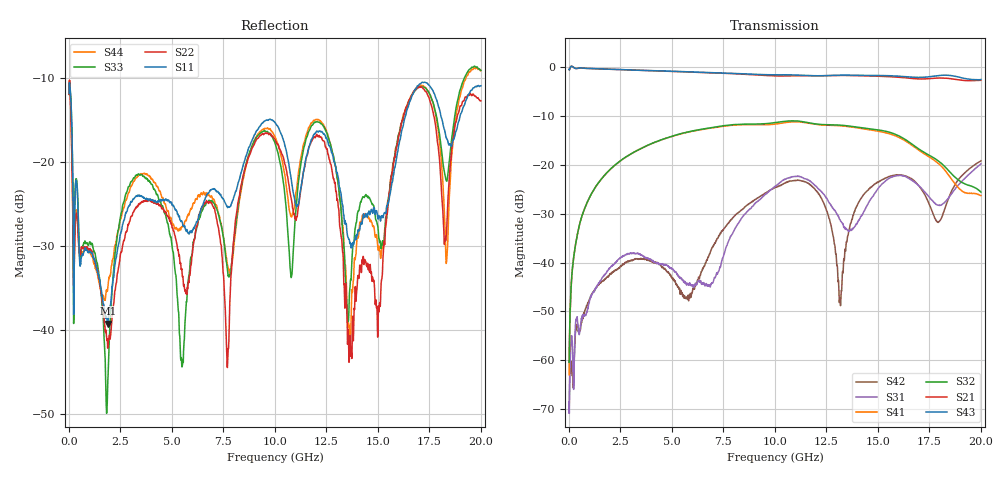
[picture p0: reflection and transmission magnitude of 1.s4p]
!Keysight Technologies,N5225A,MY51451420,A.10.40.12
!Date: Tuesday, October 13, 2015 10:13:44
!Correction: S11(Full 4 Port(1,2,3,4))
!S12(Full 4 Port(1,2,3,4))
!S13(Full 4 Port(1,2,3,4))
!S14(Full 4 Port(1,2,3,4))
!S21(Full 4 Port(1,2,3,4))
!S22(Full 4 Port(1,2,3,4))
!S23(Full 4 Port(1,2,3,4))
!S24(Full 4 Port(1,2,3,4))
!S31(Full 4 Port(1,2,3,4))
!S32(Full 4 Port(1,2,3,4))
!S33(Full 4 Port(1,2,3,4))
!S34(Full 4 Port(1,2,3,4))
!S41(Full 4 Port(1,2,3,4))
!S42(Full 4 Port(1,2,3,4))
!S43(Full 4 Port(1,2,3,4))
!S44(Full 4 Port(1,2,3,4))
!S4P File: Measurements: <S11,S12,S13,S14>,
!<S21,S22,S23,S24>,
!<S31,S32,S33,S34>,
!<S41,S42,S43,S44>:
# Hz S  dB  R 50
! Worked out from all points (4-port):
!   1999 points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, 20 MHz to 20 GHz, reference 50 ohm
!   strongest paths, dB at 20 MHz, 5.01 GHz, 10.01 GHz, 15.01 GHz, 20 GHz:
!     S43: -0.5, -0.9, -1.6, -1.7, -2.5
!     S21: -0.5, -0.9, -1.8, -1.9, -2.7
!     S32: -60.4, -14.2, -11.4, -12.9, -25.6
!     S41: -62.9, -14.2, -11.7, -13.1, -26.3
!     S31: -68.5, -41.3, -24.4, -24.9, -19.8
!     S42: -70.8, -43.1, -24.6, -23.5, -19.2
!   lowest |S11| = -39.2 dB at 1.89 GHz (marker M1), VSWR 1.02, Z = 49.7 - j1.04 ohm
!   |S11| at or under -10 dB: start of sweep to end of sweep
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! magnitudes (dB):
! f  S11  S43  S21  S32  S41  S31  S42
! 20 MHz  -11.8  -0.5  -0.5  -60.4  -62.9  -68.5  -70.8
! 1.89 GHz  -39.2  -0.4  -0.4  -21.4  -21.5  -41.6  -42.8
! 3.08 GHz  -24.7  -0.6  -0.6  -17.6  -17.6  -38.1  -39.6
! 5.5 GHz  -27.1  -0.9  -1.0  -13.6  -13.6  -43.5  -46.1
! 9.6 GHz  -15.0  -1.6  -1.7  -11.6  -11.8  -25.9  -25.7
! 13.61 GHz  -29.2  -1.7  -1.7  -12.1  -12.2  -33.5  -33.2
! 20 GHz  -10.9  -2.5  -2.7  -25.6  -26.3  -19.8  -19.2
